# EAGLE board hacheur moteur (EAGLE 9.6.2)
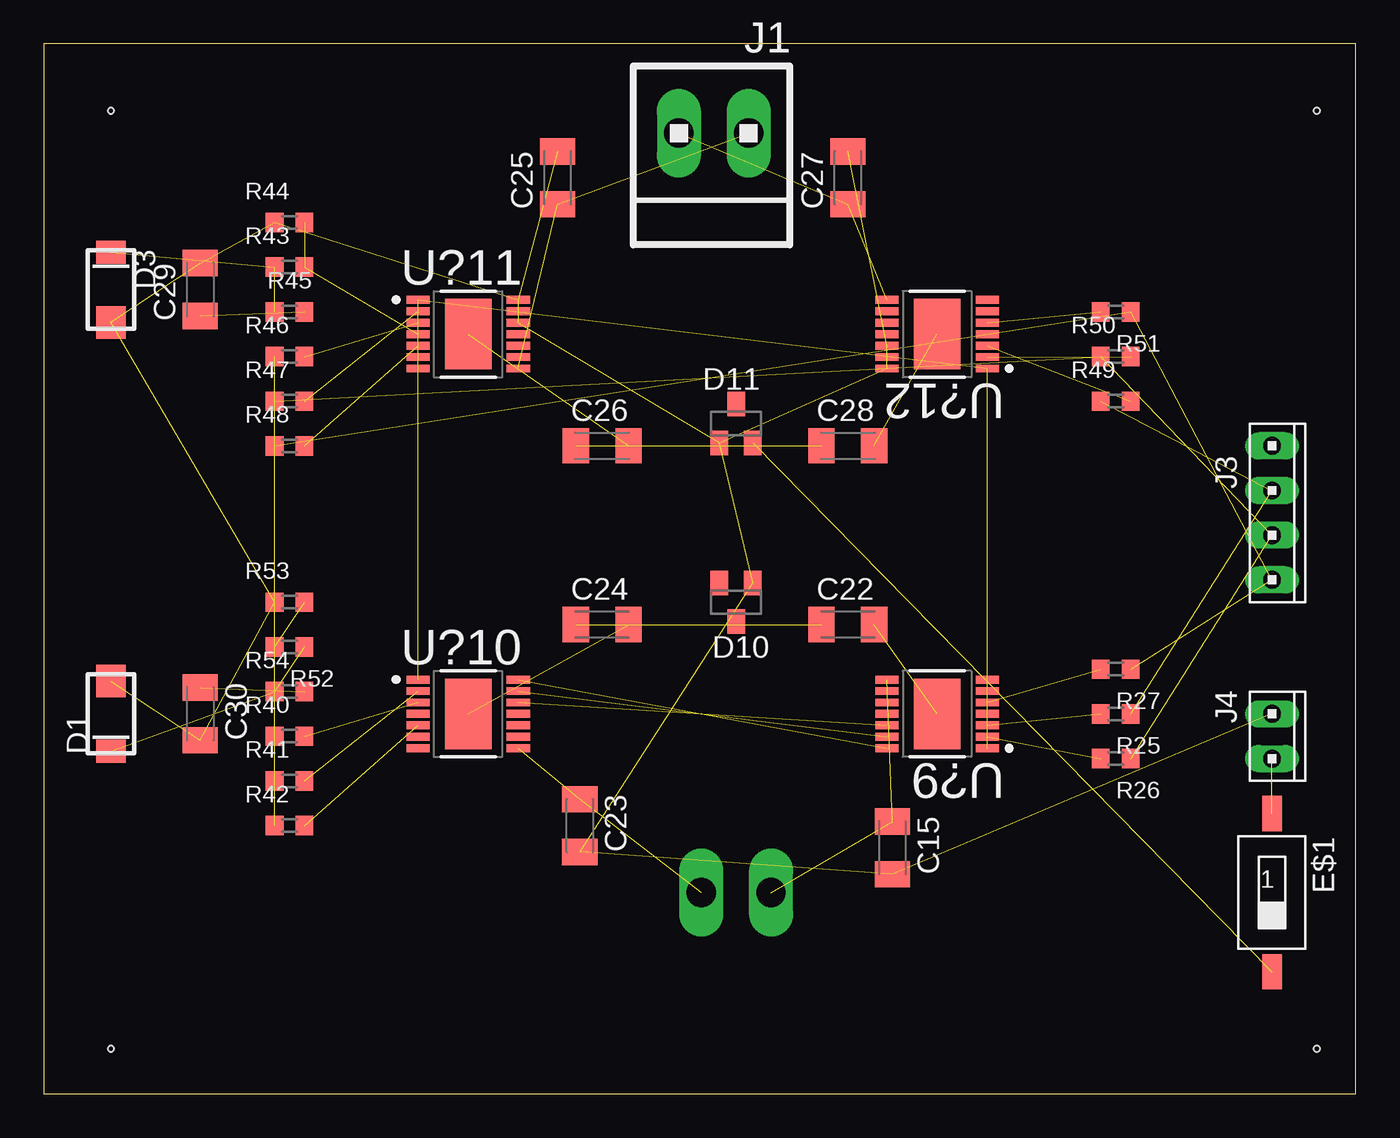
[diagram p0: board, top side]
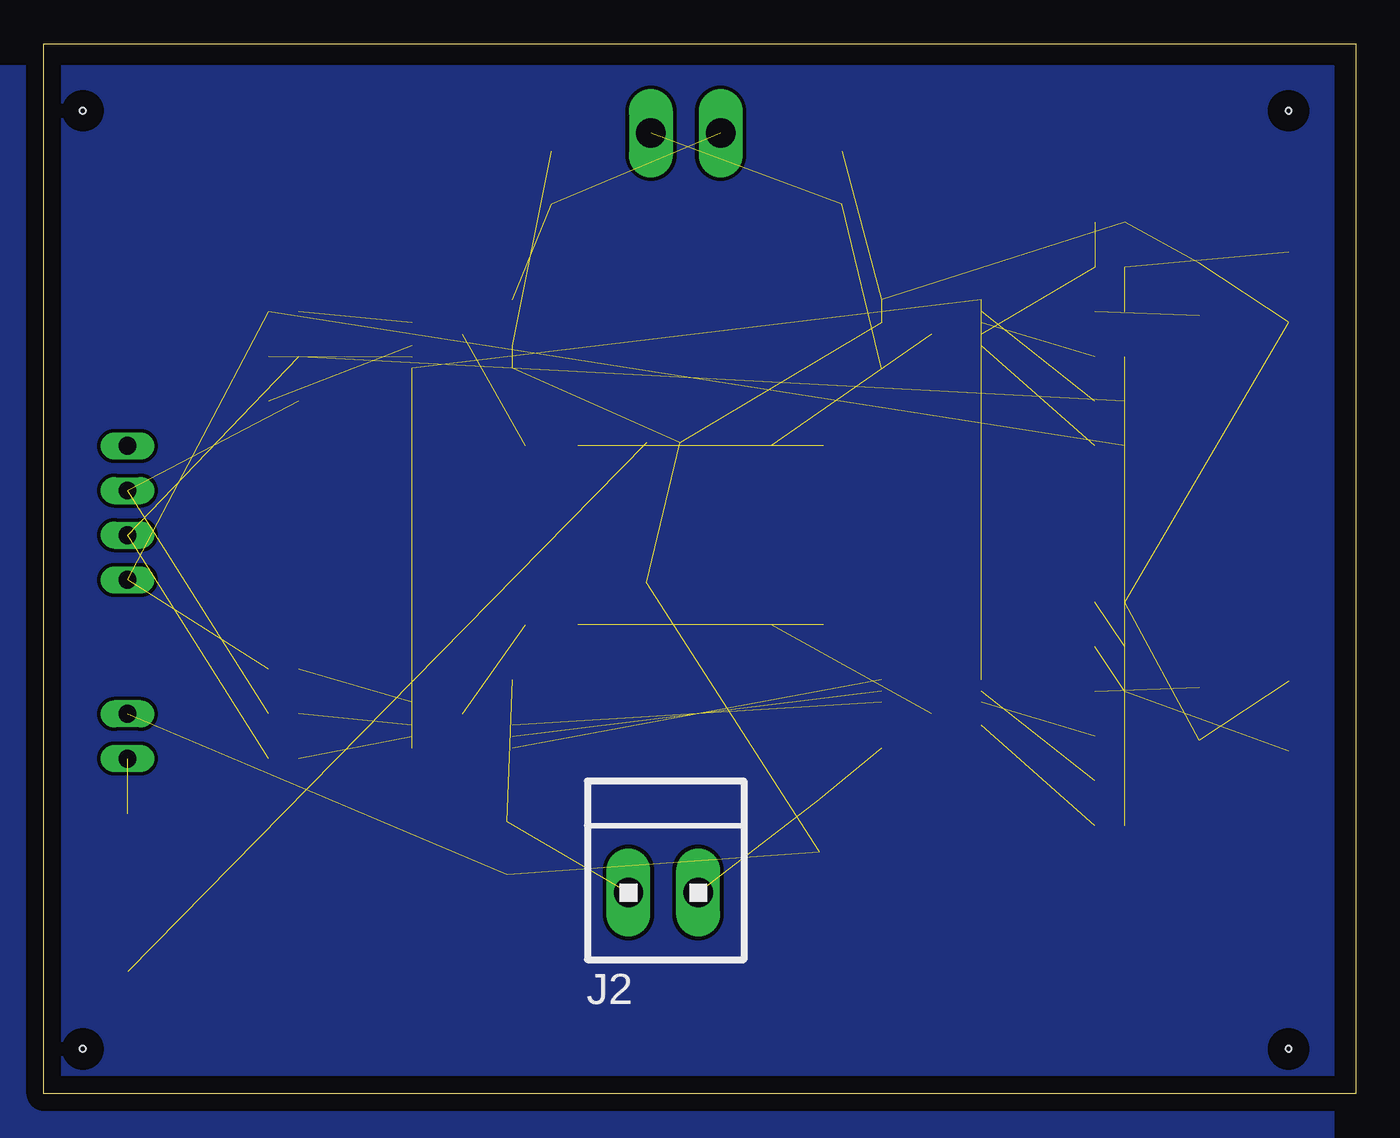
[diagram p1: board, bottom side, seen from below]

Size 74.6 x 59.68 mm. Coordinates in mm from the lower left corner, seen from the top.
Outline: 0,0 74.6,0 74.6,59.68 0,59.68 0,0
Copper layers (1*16): Top 0.035mm / dielectric 1.5mm / Bottom 0.035mm
Design rules "design rules": minimum track width 0.2mm, minimum drill 0.6mm, track to track 0.2mm, track to pad 0.2mm, pad to pad 0.185mm, via to via 0.2mm, smd to smd 0.185mm, copper to edge 1mm, drill to drill 0.4mm, minimum pad ring 0.2mm, minimum via ring 0.2mm, stop-mask expansion 4mil, vias tented up to drill 0mil, thermal gap 0.4mm
Net classes: 0 default: clearance 0.205 mm
Holes 0.35 mm at 72.39,2.54 3.81,2.54 3.81,55.88 72.39,55.88

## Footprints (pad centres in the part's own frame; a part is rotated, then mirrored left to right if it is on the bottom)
C1206K = smd 1.5 x 2: 1 -1.5,0; 2 1.5,0
GF1 = smd 1.85 x 1.68: A 1.87,0 | smd 1.32 x 1.68: C -2.12,0
SOT23C = smd 1 x 1.4: 1 -0.95,-1.1; 2 0.95,-1.1; 3 0,1.1
SMS-001 = smd 1.092 x 2.007: 1 0,-4.496; 2 0,4.496
1X2MTA = drill 1.676 long: 1 1.981,0; 2 -1.981,0
10X04MTA = drill 1.016 long: 1 3.81,0; 2 1.27,0; 3 -1.27,0; 4 -3.81,0
10X02MTA = drill 1.016 long: 1 1.27,0; 2 -1.27,0
R0603 = smd 1 x 1.1: 1 -0.85,0; 2 0.85,0
SOP65P600X115-15N-V = smd 1.31 x 0.45: 1 -2.85,1.95; 2 -2.85,1.3; 3 -2.85,0.65; 4 -2.85,0; 5 -2.85,-0.65; 6 -2.85,-1.3; 7 -2.85,-1.95; 8 2.85,-1.95; 9 2.85,-1.3; 10 2.85,-0.65; 11 2.85,0; 12 2.85,0.65; 13 2.85,1.3; 14 2.85,1.95 | smd 2.65 x 4: 15 0,0

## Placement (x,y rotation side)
C15  [C1206K]  48.26,13.97 270 top
C22  [C1206K]  45.72,26.67 0 top
C23  [C1206K]  30.48,15.24 270 top
C24  [C1206K]  31.75,26.67 0 top
C25  [C1206K]  29.21,52.07 90 top
C26  [C1206K]  31.75,36.83 0 top
C27  [C1206K]  45.72,52.07 90 top
C28  [C1206K]  45.72,36.83 0 top
C29  [C1206K]  8.89,45.72 90 top
C30  [C1206K]  8.89,21.59 270 top
D1  1N821  [GF1]  3.81,21.59 90 top
D3  1N821  [GF1]  3.81,45.72 270 top
D10  [SOT23C]  39.37,27.94 180 top
D11  [SOT23C]  39.37,38.1 0 top
E$1  [SMS-001]  69.85,11.43 180 top
J1  [1X2MTA]  38.1,54.61 180 top
J2  [1X2MTA]  39.37,11.43 0 bottom
J3  [10X04MTA]  69.85,33.02 270 top
J4  [10X02MTA]  69.85,20.32 270 top
R25  [R0603]  60.96,21.59 180 top
R26  [R0603]  60.96,19.05 180 top
R27  [R0603]  60.96,24.13 180 top
R40  [R0603]  13.97,20.32 0 top
R41  [R0603]  13.97,17.78 0 top
R42  [R0603]  13.97,15.24 0 top
R43  [R0603]  13.97,46.99 0 top
R44  [R0603]  13.97,49.53 0 top
R45  [R0603]  13.97,44.45 0 top
R46  [R0603]  13.97,41.91 0 top
R47  [R0603]  13.97,39.37 0 top
R48  [R0603]  13.97,36.83 0 top
R49  [R0603]  60.96,39.37 0 top
R50  [R0603]  60.96,41.91 0 top
R51  [R0603]  60.96,44.45 180 top
R52  [R0603]  13.97,25.4 180 top
R53  [R0603]  13.97,27.94 0 top
R54  [R0603]  13.97,22.86 0 top
U?9  [SOP65P600X115-15N-V]  50.8,21.59 180 top
U?10  [SOP65P600X115-15N-V]  24.13,21.59 0 top
U?11  [SOP65P600X115-15N-V]  24.13,43.18 0 top
U?12  [SOP65P600X115-15N-V]  50.8,43.18 180 top

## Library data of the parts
C15 C22-C30 = rcl; SPICEPREFIX: C
D1 D3 = diode
D10 D11 = semicon-smd-ipc
E$1 = smd-special
J1-J4 = con-amp
R25-R27 R40-R54 = rcl; SPICEPREFIX: R
U?9-U?12 = BTN7030-1EPA

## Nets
0: C15.2 C23.2 C25.2 C27.2 C29.2 C30.2 D1.A D3.A D10.1 D11.1 J4.2 R44.1 R53.1 U?11.12 U?11.13 U?11.14 U?12.12 U?12.13 U?12.14
GND: U?9.1 U?10.1 U?11.1 U?12.1
N$1: R48.2 U?11.5
N$2: R47.2 U?11.2
N$3: D3.C R43.1 R45.1
N$4: J3.3 R25.1 R49.1
N$91: C22.2 U?9.15
N$92: C15.1 J2.2 U?9.8
N$93: C23.1 J2.1 U?10.8
N$94: C24.2 U?10.15
N$95: C22.1 C24.1
N$96: R25.2 U?9.3
N$97: R26.2 U?9.2
N$98: R27.2 U?9.5
N$99: R40.2 U?10.3
N$100: R41.2 U?10.2
N$101: R42.2 U?10.5
N$102: C26.2 U?11.15
N$103: C25.1 J1.2 U?11.8
N$104: C27.1 J1.1 U?12.8
N$105: C28.2 U?12.15
N$106: C26.1 C28.1
N$107: R43.2 R44.2 U?11.4
N$109: C29.1 R45.2
N$110: U?12.4
N$112: R46.2 U?11.3
N$113: R51.2 U?12.5
N$114: R50.2 U?12.2
N$115: R49.2 U?12.3
N$118: R40.1 R46.1
N$119: J3.2 R26.1 R41.1 R47.1 R50.1
N$120: J3.1 R27.1 R42.1 R48.1 R51.1
N$121: U?10.4
N$122: R52.2 R53.2
N$123: D1.C R52.1 R54.1
N$124: C30.1 R54.2
N$126: J3.4
PGND_1: U?9.12 U?10.12
PGND_2: U?9.13 U?10.13
PGND_3: U?9.14 U?10.14
S$1: D11.2 E$1.2
S$2: E$1.1 J4.1

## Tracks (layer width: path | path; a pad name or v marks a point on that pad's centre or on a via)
0  (18 unrouted)
GND  (3 unrouted)
  pour Bottom: 1.27,58.42 99.06,58.42 99.06,-19.05 1.27,-19.05
N$1  (1 unrouted)
N$2  (1 unrouted)
N$3  (2 unrouted)
N$4  (2 unrouted)
N$91  (1 unrouted)
N$92  (2 unrouted)
N$93  (2 unrouted)
N$94  (1 unrouted)
N$95  (1 unrouted)
N$96  (1 unrouted)
N$97  (1 unrouted)
N$98  (1 unrouted)
N$99  (1 unrouted)
N$100  (1 unrouted)
N$101  (1 unrouted)
N$102  (1 unrouted)
N$103  (2 unrouted)
N$104  (2 unrouted)
N$105  (1 unrouted)
N$106  (1 unrouted)
N$107  (2 unrouted)
N$109  (1 unrouted)
N$112  (1 unrouted)
N$113  (1 unrouted)
N$114  (1 unrouted)
N$115  (1 unrouted)
N$118  (1 unrouted)
N$119  (4 unrouted)
N$120  (4 unrouted)
N$122  (1 unrouted)
N$123  (2 unrouted)
N$124  (1 unrouted)
PGND_1  (1 unrouted)
PGND_2  (1 unrouted)
PGND_3  (1 unrouted)
S$1  (1 unrouted)
S$2  (1 unrouted)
